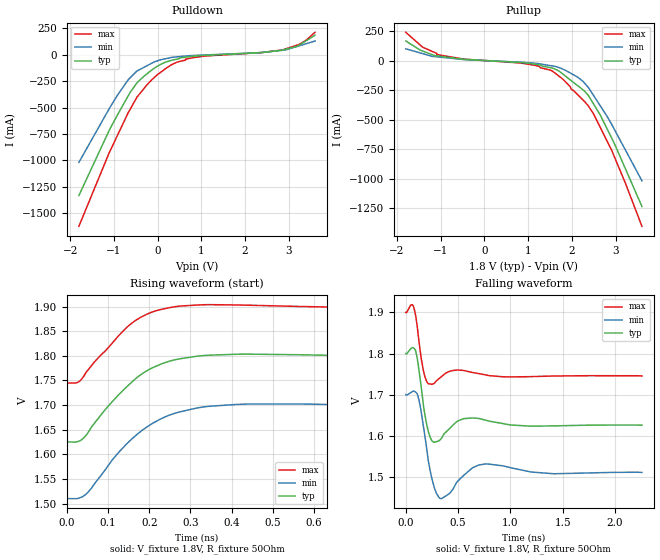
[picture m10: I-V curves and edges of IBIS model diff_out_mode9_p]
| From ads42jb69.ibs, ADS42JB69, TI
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|   diff_out_mode9 Model
[Model]   diff_out_mode9_p
Model_type   Output
Polarity   Non-Inverting
Vmeas = 1.718
Vref = 1.8
Cref = 0.5pF
Rref = 50
|   typ   min   max
|   (nom PVT)   (fast PVT)   (slow PVT)
C_comp   2.486e-12   2.313e-12   2.591e-12
[Model spec]
|subparameter   typ   min   max
Vmeas   1.728   1.618   1.816
| Where nom  PVT is Nominal Process, 1.8V, 25C
|   Fast PVT is Strong Process,  1.9V, -40C
|   Slow PVT is Weak Process,   1.7V, 125C
[Voltage Range]   1.8   1.7   1.9
[Temperature Range]   25   125   -40
[Pullup Reference]   1.8   1.7   1.9
[Pulldown Reference]   0   0   0
[Power Clamp Reference]   1.8   1.7   1.9
[GND Clamp Reference]   0   0   0
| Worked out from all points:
|   slope of the pulldown table from 0 to 0.27 V, typ, clamps not added: 5.52 ohm
|   slope of the pullup table from 0 to 0.27 V, typ, clamps not added: 49.4 ohm
|   falling waveform, V_fixture 1.8V, R_fixture 50Ohm: 20-80 % time 53.7ps typ, 65.3ps min, 48ps max; typ from 1.8 V to 1.63 V
|   rising waveform, V_fixture 1.8V, R_fixture 50Ohm: 20-80 % time 121ps typ, 132ps min, 106ps max; typ from 1.63 V to 1.8 V
[Pulldown]
|   Voltage   I(typ)   I(min)   I(max)
-1.8V     -1.331A    -1.018A    -1.622A
-1.111V   -720mA     -514.8mA   -931.9mA
-918mV    -569.7mA   -383.7mA   -763.2mA
-631.8mV  -359.5mA   -220.5mA   -519.9mA
-473.1mV  -267.8mA   -155.3mA   -402.7mA
-231.8mV  -177.9mA   -102.7mA   -280.6mA
11.97fV   -108.8mA   -57.69mA   -188.4mA
334.4mV   -51.59mA   -25.69mA   -92.26mA
642.2mV   -23.56mA   -13.7mA    -42.52mA
2.867V    43.54mA    41.82mA    45.37mA
3.228V    86.12mA    81.69mA    94.6mA
3.6V      183.6mA    128.1mA    210.7mA
[Pullup]
|   Voltage   I(typ)   I(min)   I(max)
-1.8V     165.7mA    99.47mA    239.3mA
-1.415V   80.7mA     58.56mA    113.4mA
-1.091V   39.43mA    31.42mA    50.77mA
1.146V    -30.94mA   -23.02mA   -40.66mA
1.55V     -64.42mA   -45.52mA   -88.66mA
1.796V    -115.7mA   -73.27mA   -159mA
2.249V    -247.6mA   -175.2mA   -333.1mA
2.376V    -296.6mA   -228.6mA   -385mA
2.498V    -371.1mA   -298.7mA   -455.6mA
2.907V    -656mA     -540.5mA   -759.9mA
3.219V    -914.5mA   -755.8mA   -1.036A
3.6V      -1.237A    -1.019A    -1.405A
[Ramp]
R_load = 50
|   typ   min   max
dV/dt_r   0.0586937/8.10592e-11  0.0758604/9.73276e-11  0.0474452/6.97051e-11
dV/dt_f   0.104113/5.33003e-11   0.113118/6.49875e-11  0.0923128/4.693e-11
[Falling Waveform]
V_fixture = 1.8V
V_fixture_min = 1.7V
V_fixture_max = 1.9V
R_fixture = 50Ohm
|   Time   V(typ)   V(min)   V(max)
0s        1.8V       1.7V       1.9V
64ps      1.814V     1.708V     1.919V
112ps     1.785V     1.7V       1.861V
170ps     1.672V     1.621V     1.757V
218ps     1.608V     1.536V     1.726V
276ps     1.584V     1.471V     1.728V
338ps     1.593V     1.447V     1.743V
506ps     1.637V     1.492V     1.76V
762ps     1.638V     1.531V     1.748V
2.258ns   1.626V     1.511V     1.746V
[Rising Waveform]
V_fixture = 1.8V
V_fixture_min = 1.7V
V_fixture_max = 1.9V
R_fixture = 50Ohm
|   Time   V(typ)   V(min)   V(max)
0s        1.626V     1.51V      1.745V
26ps      1.626V     1.511V     1.746V
48ps      1.641V     1.521V     1.768V
110ps     1.707V     1.589V     1.826V
148ps     1.739V     1.624V     1.86V
178ps     1.761V     1.646V     1.878V
248ps     1.789V     1.679V     1.898V
340ps     1.801V     1.697V     1.904V
444ps     1.803V     1.702V     1.903V
2.036ns   1.8V       1.7V       1.9V
